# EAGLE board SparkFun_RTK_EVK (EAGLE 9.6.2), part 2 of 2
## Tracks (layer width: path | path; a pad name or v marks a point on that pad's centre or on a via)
3.3_SW
  cutout Route15: 93.54,72.77 93.41,72.77 93.03,72.39 93.03,69.72 93.66,69.09 94.68,68.07 95.95,68.07 96.96,67.06 96.96,65.79 96.96,55.63 97.73,54.86 98.49,54.1 101.03,54.1 106.11,54.1 106.62,53.59 128.46,31.75 129.22,31.75 129.73,31.75 130.11,32.13 130.11,32.77 129.6,33.27 129.22,33.27 106.87,55.63 105.09,55.63 99.25,55.63 98.74,56.13 98.49,56.39 98.49,57.91 98.49,67.82 97.47,68.83 96.58,69.72 95.82,69.72 95.19,69.72 94.81,70.1 94.68,70.23 94.68,70.99 94.68,72.01 94.17,72.52 93.92,72.77
3.3V  (via drill 0.3)
  Top 0.406: C25.1 v68.9,24.77 | C26.1 v70.55,24.77 | v72.71,24.64 U9.14 v72.71,26.67 | C1.1 87.74,29.63 R3.2 | VID2.1 92.56,29.63 v92.52,29.59 | v108.27,28.07 108.27,27.09 C3.1 C4.1 108.31,24.42 v108.27,24.38 U2.16 | U2.4 v112.08,18.8 | v82.99,31.37 83.97,31.37 C2.1 84.05,31.37 v85.03,31.37 86,31.37 C1.1 | C1.1 85.86,31.51 U1.2
  Top 0.61: U6.5 52.7,26.77
  Top 0.813: 52.7,26.77 C14.1 C15.1 52.6,23.71 3V3.1
  Route15 0.61: v72.71,24.64 72.71,24.77
  Route15 0.813: 3V3.1 53.02,22.86 55.69,25.53 65.85,25.53 66.61,24.77 v68.9,24.77 v70.55,24.77 72.71,24.77 v72.71,26.67 77.28,26.67 81.98,31.37 v82.99,31.37 90.74,31.37 v92.52,29.59 106.74,29.59 v108.27,28.07 v108.27,24.38 108.27,19.68 109.16,18.8 v112.08,18.8
  Bottom 0.152: I2C.2 75.88,21.46 v72.71,24.64
  cutout Route15: 22.8,91.06 arc-90 24.7,89.15 arc-90 22.8,87.25 arc-90 20.89,89.15 arc-90
3.3V_SW  (via drill 0.3)
  Top 0.152: U15.23 133.03,20.49 v132.99,20.45
  Top 0.305: v129.1,23.62 U15.15 | v136.97,22.1 136.44,22.63 U15.29 | U15.36 136.94,26.13 v136.97,26.16 | v132.98,28.07 v132.99,28.07 133.03,28.02 U15.5 | U15.10 129.13,26.13 v129.1,26.16 | U7.28 59.73,73.68 v59.75,73.66
  Top 0.406: C32.1 v59.75,73.66
  Top 0.61: U3.5 57.78,27.53 | 3V3_SW.1 58.1,22.86 58.1,19.05 63.69,13.46 76.38,13.46 | J4.2 76.38,13.46 | C56.1 81.34,14.35 80.45,13.46 76.38,13.46
  Top 0.813: 57.78,27.53 C6.1 C7.1 57.68,24.98 3V3_SW.1 50.9,18.2 C19.1 C20.1 C18.1 | J3.4 46.89,13.88 46.42,14.35 C18.1 | C18.1 45.81,18.2 44.11,19.9 R11.2 R65.2 | v124.52,24.51 R18.2 | C5.1 v76.77,66.55 | C62.1 v76.77,64.9 v76.77,66.55 | U5.22 78.58,68.86 78.58,67.91 78.42,67.76 | v41.48,88.39 C52.1 | C55.1 v41.48,86.74 v41.48,88.39 | R30.2 v51.75,84.58 | R31.2 v53.53,84.58 | R32.2 v55.31,84.58 | C21.1 C32.1 | FB2.1 v43.37,67.31 v42.74,67.31 | R64.2 v76.77,75.18 | R28.2 104.2,82.46 104.46,82.21 v104.46,82.17 | v115.13,82.17 v113.47,82.17 C29.1 | v116.78,82.17 v115.13,82.17 | C30.1 v115.13,82.17 | C24.1 v116.78,82.17 | U4.36 118.68,72.14 | 118.68,72.14 118.68,74.3 | 118.68,74.3 118.68,81.28 117.79,82.17 v116.78,82.17 | U4.38 118.64,74.33 118.68,74.3 | U4.33 118.3,68.83 118.68,69.22 118.68,69.98 | 118.68,69.98 118.68,72.14 | U4.34 118.64,69.94 118.68,69.98 | R57.1 v72.83,46.61 | R54.1 69.91,39.79 v69.91,40.89 | v76.77,66.55 77.98,67.76 78.42,67.76 | 78.42,67.76 U5.23 | v96.71,73.28 95.61,73.28 C12.1 92.06,73.24 U5.7 | J13.7 41.48,95.56 v41.48,88.39
  Bottom 0.152: I2C1.2 v110.17,86.49
  pour Route15 (isolate 0.203, rank 3): 4.76,0 4.76,50.42 17.59,50.42 18.1,50.93 18.73,51.56 18.73,52.45 18.73,78.87 17.34,80.26 14.92,82.68 14.92,83.82 14.92,84.2 14.41,84.71 13.65,85.47 13.65,90.04 13.65,93.09 12.26,94.49 11.62,95.12 8.45,95.12 4.76,95.12 4.76,101.6 147,101.6 147,0
  cutout Route15: 118.43,75.95 118.43,76.58 118.05,76.96 117.54,76.96 117.28,76.71 113.35,72.77 113.35,71.37 113.35,50.04 116.27,47.12 131.64,31.75 132.02,31.75 133.03,31.75 133.41,32.13 133.41,32.77 132.78,33.4 132.65,33.53 132.52,33.53 115.13,50.93 115.13,52.2 115.13,72.01 115.89,72.77 118.43,75.31
  cutout Route15: 133.03,59.31 132.65,59.31 132.27,58.93 132.27,58.42 132.91,57.78 134.43,56.26 134.43,55.37 134.43,32.13 134.81,31.75 136.21,31.75 136.46,31.75 136.84,32.13 136.84,32.89 136.46,33.27 136.46,33.91 136.46,57.28 135.7,58.04 134.43,59.31
3.3V_SW2  (via drill 0.3)
  Top 0.152: U16.15 121.96,46.89 122.62,46.23 126.68,46.23 127.06,46.61 127.06,52.45 127.95,53.34 130.49,53.34 131.14,53.99 U18.5 134.07,54.93 135.41,53.59 v140.65,53.59
  Top 0.406: U12.1 60.94,28.41 61.02,28.32
  Top 0.813: 3V3_SW2.1 61.06,23.71 C61.1 C60.1 61.06,28.28 61.02,28.32 | v141.92,53.59 v140.65,53.59 | v141.92,53.59 v143.19,53.59 | 140.14,82.3 140.14,83.19 139.94,83.39 U8.53 C80.1 C79.1 138.75,88.94 C81.1 140.44,88.9 C78.1 142.04,88.85 C77.1 141.92,87.01 C76.+ v141.92,53.59 | 140.14,82.3 140.14,81.41 139.93,81.19 U8.51 | U8.52 140.14,82.29 140.14,82.3
  Route15 0.813: v140.65,53.59 v141.92,53.59 v143.19,53.59 144.46,52.32 144.46,20.32 140.65,16.51 126.68,16.51 122.62,12.45 108.52,12.45 106.36,14.61 99.38,14.61 91.16,22.82 61.95,22.82 3V3_SW2.1
5V
  Top 0.152: U6.3 50.8,32.96 51.24,33.4 52.7,33.4
  Top 0.406: U12.8 60.94,32.55 61.02,32.64
  Top 0.61: U6.1 52.7,33.4 | U3.1 57.78,34.19
  Top 0.813: 52.7,33.4 52.7,34.19 C17.1 R51.2 R50.2 52.6,38.95 54.29,40.64 5V.1 | 57.78,34.19 C9.1 C8.1 C10.1 | 5V.1 57.68,40.22 C10.1 | C10.1 C23.1 C22.1 C59.1 61.06,32.68 61.02,32.64 | R59.1 F1.1 54.78,53.71 R53.1 | R59.1 57.97,48.13 56.69,46.85 C57.+ | C57.+ 56.69,43.32 58.1,41.91 5V.1 | 5V.1 58.14,40.68 60.26,40.68 C53.1 60.74,40.96 U13.5 | C57.+ 58.86,44.45 59.28,44.87 C54.1 60.74,44.77 U11.5 | R59.1 R55.1 R60.1 R61.1
5V_RAW
  Top 0.813: U10.2 U10.1 29.72,54.17 30.3,54.75 C48.+ 32.93,54.98 C49.1 | C49.1 C50.1 | L1.1 37.78,53.38 C49.1
5V_RAW1
  Top 0.813: C16.+ 41.96,26.9 C51.1 C84.1 42.06,33.63 L4.1
  Top 1.905: U17.4 C16.+
9%  (via drill 0.3)
  Top 0.152: 9%.1 50.48,58.42 53.87,58.42 | R48.2 53.87,58.42 | 53.87,58.42 R58.1 | U13.3 64.77,42.86 v63.94,43.69
  Bottom 0.152: v63.94,43.69 61.91,45.72 61.91,47.62 56.2,53.34 47.94,53.34 9%.1
99%  (via drill 0.3)
  Top 0.152: 99%.1 R53.2 R48.1 | U11.4 62.52,47.47 v62.55,47.5
  Bottom 0.152: v62.55,47.5 56.32,53.72 50.1,53.72 99%.1
!ANT_SHORT!  (via drill 0.3)
  Top 0.152: Q2.6 70.15,46.41 R57.2 69.95,47.41 ANT_SHT.1 | v78.6,48.26 78.72,48.39 v78.72,64.36 | v100.14,72.14 U4.6
  Bottom 0.152: ANT_SHT.1 v78.6,48.26 | v100.14,72.14 100.14,67.69 97.06,64.61 78.98,64.61 v78.72,64.36
!RESET!  (via drill 0.3)
  Top 0.152: U7.37 58.8,79.18 59.12,79.5 59.12,83.58 60.37,84.84 64.65,84.84 67.12,82.37 67.12,77.67 v67.32,77.47 67.12,77.27 67.12,57.02 v68.26,55.88 | v87.19,35.33 87.13,35.28 U1.3 87.13,32.95 87.95,32.13 R3.1 C31.1 91.12,30.06 91.12,27.94 v94.93,24.13 | U9.12 v75.25,35.31 74.87,35.69 v68.26,35.69 | v99.76,21.21 99.79,21.24 Q1.3
  Bottom 0.152: v67.32,77.47 GNSS_RESET.4 GNSS_RESET.2 | v87.19,35.33 75.28,35.33 v75.25,35.31 | v68.26,55.88 v68.26,35.69 | RESET_SW.1 101.28,12.7 98.74,15.24 98.74,20.19 v99.76,21.21 96.84,24.13 v94.93,24.13
!SAFEBOOT_NEO!
  Top 0.152: U5.1 94.06,66.66 94.68,66.04 !SAFEBOOT_NEO!.1
!SAFEBOOT_ZED!
  Top 0.152: U4.50 106.83,80.56 106.83,87.16 !SAFEBOOT_ZED!.1
ACT
  Bottom 0.152: ACT.1 9.07,98.16 8.29,97.38 J9.14
ACT_LED
  Top 0.152: U7.27 59.34,73.18 59.75,72.77 59.75,70.23 60.13,69.85 R26.2
ANT
  Top 0.349: C13.2 U14.2
ANT_DET  (via drill 0.3)
  Top 0.152: Q2.3 71.45,39.95 R54.2 71.65,38.95 ANT_DET.1 | v79.69,65.41 v79.69,38.1 | U4.4 100.05,74.33 99.63,73.91 v99.63,71.63
  Bottom 0.152: v99.63,71.63 99.63,67.7 96.82,64.89 80.2,64.89 v79.69,65.41 | v79.69,38.1 ANT_DET.1
ANT_NEO
  Top 0.318: 92.1,79.5 arc-90 U5.11
  Top 0.349: U14.5 94.93,81.03 arc-90 93.41,79.5 92.1,79.5
ANT_ZED
  Top 0.318: 101.41,76.58 arc-90 U4.2
  Top 0.349: U14.8 98.74,78.23 arc90 100.39,76.58 101.41,76.58
BYPASS
  Top 0.349: BYPASS1.1 97.47,85.72 arc90 98.11,85.09 arc-90 98.74,84.45 BYPASS2.1
CH340-DTR  (via drill 0.3)
  Top 0.152: R4.2 103.75,21.24 v102.81,21.24 Q1.1 101.93,22.21 101.28,22.86 DTR.1 | U2.13 112.08,21.84 111.44,21.21 v106.36,21.21
  Bottom 0.152: v106.36,21.21 102.84,21.21
  Bottom 0.267: 102.84,21.21 v102.81,21.24
CH340-RTS  (via drill 0.3)
  Top 0.152: R5.2 98.81,19.4 v99.76,19.4 Q1.4 100.63,18.43 101.28,17.78 RTS.1 | U2.14 110.81,22.23 110.43,21.85 105.99,21.85 105.22,21.08 v105.22,19.43
  Bottom 0.152: 105.19,19.4 v99.76,19.4
  Bottom 0.267: v105.22,19.43 105.19,19.4
CH340-RXI  (via drill 0.3)
  Top 0.152: TX.1 110.81,15.88 U2.3 v110.81,19.94 | v94.93,47.62 94.81,47.5 92.7,47.5 88.4,51.8 U1.35
  Bottom 0.152: v110.81,19.94 109.28,19.94 109.03,20.19 109.03,35.01 96.41,47.62 v94.93,47.62
CH340-TXO  (via drill 0.3)
  Top 0.152: RX.1 109.54,15.88 U2.2 v109.54,20.57 | v94.93,48.54 92.93,48.54 89.67,51.8 U1.34
  Bottom 0.152: v109.54,20.57 109.54,34.9 95.89,48.54 v94.93,48.54
D+  (via drill 0.3)
  Top 0.152: 113.73,8.89 J1.A6 113.73,5.33 113.98,5.08 114.49,5.08 114.73,5.32 J1.B6
  Top 0.267: 113.73,8.89 113.03,9.59 D10.1 113.03,11.37 v113.22,11.56 | v113.47,16.51 113.47,16.63 113.35,16.76 U2.5
  Bottom 0.267: v113.47,16.51 113.73,16.26 113.73,12.06 v113.22,11.56
D+_LARA
  Top 0.267: U15.2 134.53,27.79 135.19,28.45 135.19,29.25 R10.1
D+_NEO
  Top 0.267: R66.1 128.59,29.25 128.59,29.08 129.86,27.81 131.64,27.81 132.03,27.42 U15.7
D+_UBLOX
  Top 0.267: J6.A6 139.13,5.2 139.26,5.08 139.89,5.08 140.13,5.32 J6.B6 140.13,7.87 141.54,9.28 141.54,10.79 140.33,12 D8.1 140.33,13.15 139.92,13.56 139.92,15.31 R23.1
D+_ZED
  Top 0.267: R7.1 131.51,29.46 132.37,28.6 133.38,28.6 133.53,28.46 U15.4
D-  (via drill 0.3)
  Top 0.152: J1.B7 113.22,6 v113.22,7.11 | 114.23,8.89 114.23,7.24 v114.36,7.11 114.23,6.98 J1.A7
  Top 0.267: 114.23,8.89 114.93,9.59 D10.3 114.93,11.37 v114.74,11.56 | v114.49,16.51 114.62,16.64 U2.6
  Bottom 0.152: v114.36,7.11 v113.22,7.11
  Bottom 0.267: v114.49,16.51 114.24,16.26 114.24,12.06 v114.74,11.56
D-_LARA
  Top 0.267: U15.1 135.03,27.65 135.7,28.32 135.7,28.87 R9.1
D-_NEO
  Top 0.267: U15.6 132.53,27.53 131.85,28.21 130.1,28.21 129.48,28.83 129.48,29.25 R67.1
D-_UBLOX
  Top 0.267: J6.A7 139.63,6.99 | 139.63,6.99 139.63,8 141.02,9.38 141.02,10.76 140.1,11.68 138.62,11.68 138.43,11.87 D8.3 138.43,13.15 138.85,13.56 138.85,15.31 R22.1 | J6.B7 138.63,6.74 138.87,6.99 139.63,6.99
D-_ZED
  Top 0.267: U15.3 134.03,28.76 R8.1
ESP0/!BOOT!  (via drill 0.3)
  Top 0.152: Q1.6 101.93,18.89 102.03,18.8 v102.55,18.8 | U1.25 101.1,42.09 v101.28,41.91
  Bottom 0.152: v102.55,18.8 105.35,18.8 105.85,19.3 107.63,19.3 | 107.63,19.3 120.08,19.3 TP_BOOT.1 BOOT_SW.1 | v101.28,41.91 101.66,41.91 107.63,35.94 107.63,19.3
ESP2/LED  (via drill 0.3)
  Top 0.152: R62.1 TP_LED.1 | v98.74,62.28 98.74,59.44 99.76,58.42 101.92,58.42 102.37,57.97 U1.24
  Bottom 0.152: TP_LED.1 14.92,13.97 14.92,17.78 20,22.86 25.97,22.86 26.5,23.39 26.5,45.03 34.12,52.65 34.12,60.15 36.05,62.08 98.54,62.08 v98.74,62.28
ESP4/!SD_CS!  (via drill 0.3)
  Top 0.152: J3.2 49.09,13.85 SD_CS.1 | U1.26 99.83,56.47 v99.76,56.54 | v76.42,28.45 76.39,28.48 76.39,55.88 76.39,56.26 76.39,56.52 v76.14,56.77 | v66.99,28.45 v66.99,16.38
  Bottom 0.152: v76.42,28.45 v66.99,28.45 | v99.76,56.54 99.66,56.64 77.66,56.64 77.28,56.26 76.64,56.26 v76.14,56.77 | v66.99,16.38 51.63,16.38 SD_CS.1
ESP5/TP
  Top 0.152: U9.8 80.33,27.3 82.23,29.21 82.23,39.37 88.58,45.72 94.93,45.72 96.02,46.81 U1.29
ESP12/SDA2
  Top 0.152: U9.4 76.52,18.92 77.03,18.41 90.49,18.41 101.1,29.03 U1.14
ESP13/LARA_TXDI  (via drill 0.3)
  Top 0.152: U1.16 103.64,36.9 104.2,37.47 v119.82,37.47 119.82,36.2 119.57,35.94 119.44,35.94 119.06,35.56 119.06,30.48 TXD.1 | v119.95,46.48 119.95,47.84 U16.12
  Bottom 0.152: v119.82,37.47 119.82,46.35 v119.95,46.48
ESP14/LARA_RXDO  (via drill 0.3)
  Top 0.152: U1.13 99.83,36.9 100.9,37.97 120.46,37.97 v120.59,37.85 120.59,32 RXD.1 | v120.71,46.48 120.71,47.84 U16.13
  Bottom 0.152: v120.59,37.85 120.59,46.35 v120.71,46.48
ESP15/SCL2  (via drill 0.3)
  Top 0.152: U1.23 103.64,56.7 v103.57,56.77 | v76.9,56.77 v76.9,27.94 | v73.34,27.94 73.34,22.86 72.71,22.23 U9.1
  Bottom 0.152: v103.57,56.77 103.31,57.02 77.15,57.02 v76.9,56.77 | v76.9,27.94 v73.34,27.94
ESP18/SCK  (via drill 0.3)
  Top 0.152: J3.5 45.79,13.58 SCK.1 | U7.33 59.85,76.18 60.24,76.57 60.24,83.05 60.91,83.72 64.19,83.72 66,81.9 66,54.08 v66.23,53.85 66.3,53.78 v75.25,53.78 | v65.98,15.42 v65.98,30.1 | v94.68,53.72 94.75,53.65 U1.30
  Bottom 0.152: SCK.1 45.68,13.69 51.87,13.69 53.6,15.42 v65.98,15.42 | v65.98,30.1 66.02,30.1 66.2,30.28 66.2,53.82 v66.23,53.85 | v75.25,53.78 75.37,53.65 94.55,53.65 94.65,53.75 v94.68,53.72
ESP19/POCI  (via drill 0.3)
  Top 0.152: J3.7 43.59,13.49 41.85,15.24 POCI.1 41.59,16.3 R11.1 | U7.34 59.8,76.68 59.96,76.83 59.96,83.16 60.79,84 64.3,84 66.28,82.02 66.28,54.76 v66.71,54.33 74.54,54.33 v74.61,54.26 | v65.47,14.94 v65.47,28.83 | v93.41,54.23 93.48,54.16 U1.31
  Bottom 0.152: POCI.1 43.47,13.36 44.84,13.36 44.89,13.41 51.98,13.41 53.52,14.94 v65.47,14.94 | v65.47,28.83 65.47,28.91 66.71,30.15 v66.71,54.33 | v74.61,54.26 93.38,54.26 v93.41,54.23
ESP21/SDA  (via drill 0.3)
  Top 0.152: U5.18 80.01,73.23 v78.55,73.23 | v68.74,56.36 67.4,57.71 67.4,72.44 v67.6,72.64 67.88,72.93 67.88,82 64.03,85.85 47.18,85.85 44.92,88.11 44.92,92.02 | U4.44 113.3,81.33 113.09,81.53 112.46,81.53 111.06,82.93 R72.1 112.17,83.61 v112.2,83.57 | v90.87,63.22 v90.87,55.5 90.94,55.42 U1.33 90.94,51.8 93.21,49.53 v94.93,49.53
  Top 0.305: D15.1 44.92,92.02 J13.6
  Bottom 0.152: SDA.1 44.92,97.31 J13.6 | v67.6,72.64 77.96,72.64 v78.55,73.23 | v68.74,56.36 75.4,56.36 76.13,55.63 90.74,55.63 v90.87,55.5 | v112.2,83.57 112.2,82.93 108.42,79.15 108.42,73.92 97.84,63.35 91,63.35 v90.87,63.22 | USB251SDA.1 126.58,18.64 95.69,49.53 v94.93,49.53
ESP22/SCL  (via drill 0.3)
  Top 0.152: U5.19 78.57,72.16 v78.55,72.14 | v69.23,56.84 67.68,58.39 67.68,71.76 v67.97,72.05 68.16,72.24 68.16,82.12 64.15,86.13 49.7,86.13 48.42,87.4 48.42,92.02 | U4.45 112.2,81.28 111.82,81.66 109.92,81.66 109.41,82.17 R71.1 108.18,83.61 v108.14,83.57 | v88.33,63.5 88.33,57.43 v87.06,56.16 87.13,56.09 U1.36 87.13,51.87 89.47,49.53 v89.85,49.53
  Top 0.305: D16.1 48.42,92.02 J13.5
  Bottom 0.152: SCL.1 48.42,98.27 J13.5 | v67.97,72.05 68.28,72.36 77.81,72.36 78.04,72.14 v78.55,72.14 | v69.23,56.84 75.38,56.84 76.32,55.91 77.43,55.91 77.79,56.26 86.96,56.26 v87.06,56.16 | v108.14,83.57 108.14,74.17 97.68,63.7 88.53,63.7 v88.33,63.5 | USB251SCL.1 134.05,18.14 133.82,17.91 126.92,17.91 95.81,49.02 90.36,49.02 v89.85,49.53
ESP23/PICO  (via drill 0.3)
  Top 0.152: J3.3 47.94,12.58 PICO.1 | U7.35 59.51,77.18 59.68,77.34 59.68,83.28 60.68,84.28 64.42,84.28 66.56,82.14 66.56,55.55 v67.25,54.86 73.92,54.86 v73.98,54.81 | v66.48,15.9 v66.48,29.21 | v85.79,54.74 85.86,54.66 U1.37
  Bottom 0.152: PICO.1 49.21,13.97 51.75,13.97 53.69,15.9 v66.48,15.9 | v66.48,29.21 67.25,29.97 v67.25,54.86 | v73.98,54.81 85.72,54.81 v85.79,54.74
ESP25/ZED_TXO  (via drill 0.3)
  Top 0.152: U4.42 116.63,80.44 v116.68,80.39 | v94.81,62.56 94.81,55.75 v96.58,53.98 | v96.58,50.29 97.98,50.29 98.74,49.53 98.74,40.01 96.02,37.28 U1.10
  Bottom 0.152: v116.68,80.39 116.68,80.28 116.75,80.21 116.75,64.12 114.98,62.36 100.03,62.36 99.35,63.04 95.29,63.04 v94.81,62.56 | v96.58,53.98 v96.58,50.29 96.58,49.4 97.09,48.9 105.73,48.9 ZED_TXO.1
ESP26/LARA_PWR_ON
  Top 0.152: U1.11 97.29,36.65 98.97,38.33 124.37,38.33 131.76,45.72 R70.1 R69.2
ESP27/!ETH_CS!  (via drill 0.3)
  Top 0.152: U7.32 59.74,75.68 60.52,76.45 60.52,82.93 61.02,83.44 64.07,83.44 65.72,81.79 v65.72,53.34 | v65.72,36.83 v75.25,36.83 | v98.49,36.83 98.49,34.25 U1.12 98.56,33.2 ETH_CS.1
  Bottom 0.152: v65.72,53.34 v65.72,36.83 | v75.25,36.83 v98.49,36.83
ESP32/PWREN  (via drill 0.3)
  Top 0.152: U9.11 76.52,25.91 78.68,28.07 v78.68,37.34 | v93.41,37.31 93.41,34.25 U1.8
  Bottom 0.152: v78.68,37.34 93.38,37.34 v93.41,37.31
ESP33/ZED_RXI  (via drill 0.3)
  Top 0.152: U4.43 114.4,81.34 114.62,81.56 116.62,81.56 v117.16,81.03 | U1.9 94.75,36.65 97.47,39.37 v97.47,49.53 | v97.47,53.98 95.57,55.88 95.57,61.95 v96.17,62.56
  Bottom 0.152: v117.16,81.03 117.16,64.14 115.1,62.08 99.78,62.08 99.1,62.76 98.38,62.76 98.23,62.61 96.23,62.61 v96.17,62.56 | v97.47,53.98 v97.47,49.53 107.63,49.53 ZED_RXI.1
ESP34/LARA_NI  (via drill 0.3)
  Top 0.152: U16.14 121.31,40.34 119.57,38.61 v98.11,38.61 | v91,37.85 90.94,37.79 U1.6
  Bottom 0.152: v91,37.85 91.76,38.61 v98.11,38.61
ESP35/VID
  Top 0.152: VID1.2 VID2.2 92.81,31.33 92.21,31.93 U1.7
ESP36/SD_DET  (via drill 0.3)
  Top 0.152: J3.9 41.39,12.9 DET.1 39.05,15.41 R65.1 | v69.02,35.18 64.96,31.11 v64.96,14.46 | U1.4 88.4,35.74 v88.33,35.81
  Bottom 0.152: DET.1 41.21,13.08 44.96,13.08 45,13.13 52.1,13.13 53.43,14.46 v64.96,14.46 | v69.02,35.18 69.66,35.81 v88.33,35.81
ESP39/!ETH_INT!  (via drill 0.3)
  Top 0.152: U7.36 58.95,77.68 59.4,78.13 59.4,83.46 60.49,84.56 64.53,84.56 66.84,82.25 66.84,56.29 v67.75,55.37 | v67.75,36.32 v75.88,36.32 | U1.5 89.67,36.27 v89.73,36.32
  Bottom 0.152: v75.88,36.32 v89.73,36.32 95.44,36.32 97.47,34.29 ETH_INT.1 | v67.75,55.37 v67.75,36.32
GND  (via drill 0.3)
  Top 0.305: v129.1,24.89 129.1,25.31 129.42,25.63 U15.11 131.53,25.63 U15.EP
  Bottom 0.152: SHLD1.1 113.97,3.68 v112.59,3.68 | SHLD2.1 139.27,3.81 v138.11,3.81
  other vias: 28.89,73.66 28.89,72.39 28.89,71.12 28.89,69.85 26.35,68.58 26.35,67.31 26.35,66.04 26.35,64.77 26.35,63.5 26.35,62.23 26.35,60.96 26.35,59.69 27.62,59.69 27.62,60.96 27.62,62.23 27.62,63.5 27.62,64.77 27.62,66.04 27.62,67.31 27.62,68.58 28.89,68.58 28.89,67.31 28.89,66.04 28.89,64.77 28.89,63.5 28.89,62.23 28.89,60.96 28.89,59.69 28.26,60.33 26.99,60.33 26.99,61.59 28.26,61.59 28.26,62.87 26.99,62.87 26.99,64.14 26.99,65.41 26.99,66.67 28.26,67.94 26.99,67.94 28.26,66.67 28.26,65.41 28.26,64.14 26.99,59.05 28.26,59.05 27.62,58.42 26.35,58.42 28.89,58.42 41.59,59.69 42.86,59.69 44.13,59.69 45.4,59.69 46.67,59.69 45.4,58.42 46.67,58.42 44.13,58.42 42.23,59.05 43.5,59.05 44.77,59.05 44.77,57.78 46.04,59.05 46.04,57.78 40.32,59.69 39.05,59.69 39.05,58.42 40.32,58.42 40.96,59.05 39.69,59.05 39.69,57.78 40.96,57.78 21.02,17.14 16.45,17.14 26.86,21.08 28.51,21.08 29.78,21.08 25.21,21.08 23.56,21.08 30.29,16 62.93,28.19 63.94,26.67 63.94,24.51 49.72,26.67 49.72,24.77 54.67,25.78 54.67,27.43 56.83,32.89 56.83,30.73 51.75,30.73 51.75,32.89 63.94,29.21 54.8,36.2 54.8,38.1 63.94,38.1 63.94,36.2 63.82,33.4 49.72,34.29 54.93,33.4 32.7,61.59 31.81,61.59 33.59,61.59 37.78,57.78 41.08,54.48 50.86,59.69 63.94,45.72 63.94,41.91 60.64,47.75 59.5,42.8 70.17,42.04 71.44,45.59 49.21,44.45 49.21,45.47 49.21,43.43 142.05,48.77 141.03,48.77 143.07,48.77 118.43,49.4 129.86,55.88 133.41,52.07 128.59,51.31 127.57,62.99 129.6,62.99 131.76,62.99 133.92,62.99 135.95,62.99 125.16,60.33 138.24,60.33 127.57,69.34 135.95,69.34 127.57,75.44 135.95,75.44 127.57,81.79 129.73,81.79 131.76,81.79 133.79,81.79 135.95,81.79 123.51,81.15 123.51,83.44 125.03,84.45 127.32,86.36 126.3,86.36 127.32,87.63 127.32,88.9 127.32,90.17 127.32,91.44 126.81,92.2 125.41,92.08 123.76,92.08 121.98,92.08 120.71,92.08 119.19,92.58 118.55,93.98 117.28,95.25 117.16,96.65 115.76,99.31 115.76,98.04 116.01,96.9 115.76,100.33 123.63,100.33 123.63,99.31 123.63,98.04 123.38,96.77 122.36,96.65 120.97,95.89 121.73,94.87 123.76,94.87 125.41,96.39 126.94,95.12 128.08,94.11 129.22,92.71 129.22,91.44 129.22,90.17 129.22,88.9 129.22,87.63 129.22,86.36 130.49,86.36 134.3,86.36 133.03,86.36 134.3,87.63 134.3,88.9 134.3,90.17 134.3,91.44 134.3,92.71 134.81,94.11 135.57,95.12 136.84,96.27 137.99,99.31 137.99,100.33 137.99,98.04 138.24,96.65 139.38,96.65 140.65,95.25 138.49,95.25 145.86,99.31 145.86,100.33 145.86,98.04 145.61,96.65 144.59,96.65 144.21,95.25 143.19,94.11 142.68,92.96 141.41,92.2 140.4,92.08 138.62,92.08 136.97,92.08 136.08,91.06 135.83,88.9 135.83,87.25 136.08,85.98 137.22,85.98 101.54,99.06 101.54,100.33 101.54,97.79 101.28,96.52 100.01,96.52 98.74,95.25 98.74,93.47 98.74,91.69 98.74,89.92 96.2,89.92 96.2,91.69 94.55,91.69 93.03,90.42 91.12,91.44 95.06,95.25 94.42,94.49 94.93,96.52 93.66,96.65 93.41,99.06 93.41,97.79 93.41,100.33 94.93,89.15 94.93,85.09 96.2,85.09 97.47,84.2 98.74,85.98 96.2,81.28 97.47,81.28 93.54,86.87 93.54,85.09 93.54,83.31 93.79,80.9 92.14,81.92 90.36,80.64 90.36,79.63 90.36,78.49 94.04,78.49 95.44,79.63 97.73,79.76 97.73,78.23 98.23,76.71 99.76,75.44 99.76,77.72 99.76,79.76 99.76,81.28 100.39,82.8 100.39,85.09 100.39,87.63 101.41,78.61 103.82,76.71 108.9,76.71 112.97,76.71 112.97,72.52 108.9,72.52 104.71,68.33 108.9,68.33 112.97,68.33 104.71,64.14 108.9,64.14 112.97,64.14 117.79,67.82 117.79,77.6 100.01,63.37 117.79,73.28 71.18,99.06 79.31,99.06 71.18,100.46 71.18,97.54 79.31,97.41 79.31,100.46 72.71,96.52 72.83,94.61 77.79,96.65 76.9,95.5 76.39,94.61 76.52,92.46 77.79,90.81 76.64,89.03 73.98,89.03 75.25,89.03 72.83,90.68 73.98,92.46 48.07,21.84 46.29,21.84 49.72,21.84 44.64,13.84 44.77,11.18 40.83,37.59 45.02,33.53 78.42,12.45 78.42,11.43 82.61,16.38 67.63,21.84 71.69,21.84 80.33,21.72 83.76,21.97 110.17,13.46 117.79,13.46 113.98,11.56 139.76,32.51 145.99,25.27 145.99,23.5 124.65,22.86 124.65,26.16 72.58,66.55 72.58,64.9 81.47,66.67 81.47,80.64 124.4,50.8 118.81,52.2 116.27,50.8 52.01,71.88 53.02,71.88 51.24,73.66 54.55,71.88 57.34,74.17 51.24,76.58 51.5,78.11 43.37,73.03 43.37,71.12 43.37,69.22 63.94,73.66 63.94,71.75 49.21,65.28 51.12,65.28 53.02,65.28 54.93,65.28 56.83,65.28 58.74,65.28 48.07,83.31 63.44,82.93 61.53,82.93 40.32,83.31 37.27,71.12 37.27,83.82 37.02,86.74 37.02,88.39 37.78,77.47 72.58,73.53 95.57,70.36 107.38,17.53 83.63,52.7 83.63,51.69 83.63,33.66 83.63,34.67 89.98,41.66 92.39,39.37 89.98,39.37 92.39,44.07 89.98,44.07 94.81,41.66 94.81,44.07 94.81,39.37 102.43,35.43 95.57,28.45 89.85,28.45 86.04,28.45 84.01,28.45 135.57,13.46 143.19,13.46 139.38,13.97 117.28,6.99 108.52,5.97 142.68,6.99 133.92,5.97 130.11,14.48 131.76,14.48 133.41,14.48 136.72,14.48 138.11,32.51 55.56,59.69 55.56,57.15 55.56,54.61 56.32,52.07 56.32,49.53 63.18,59.69 63.18,57.15 69.53,60.45 73.34,60.45 77.15,60.45 82.23,60.45 84.77,60.45 70.8,58.67 73.34,58.67 75.88,58.67 78.17,58.67 81.6,58.67 83.5,58.67 86.04,58.67 84.77,63.37 87.31,60.45 87.31,63.37 84.77,67.31 87.31,67.31 87.31,69.85 84.77,69.85 84.77,72.39 84.77,74.93 84.77,78.74 84.77,81.28 87.31,72.39 87.31,74.93 87.31,78.74 87.31,81.28 84.77,83.82 84.77,86.36 84.77,88.9 84.77,91.44 86.04,93.98 88.58,94.61 91.12,94.61 87.31,83.82 87.31,86.36 87.31,88.9 88.58,91.44 103.82,74.68 103.82,78.87 100.01,64.77 135.57,58.67 123.51,69.09 145.1,88.9 144.97,87.12 108.9,81.79 113.47,86.61 115,86.61 116.78,86.61 140.02,80.01 123.51,78.99 123.51,74.55 123.51,73.53 140.02,72.39 123.51,62.48 111.32,27.05 111.32,25.4 106.87,76.71 104.71,72.64 128.46,14.48 126.81,14.48 46.67,89.79 50.23,89.79 53.66,89.79 57.21,89.79 60.64,89.79 64.33,89.79 125.41,55.88 133.03,24.13 84.77,48.26 86.04,48.26 14.92,87.63 17.46,87.63 14.92,90.17 23.81,83.82 32.7,83.82 31.43,74.93 26.35,74.93 26.35,77.47 31.43,77.47 28.89,77.47 20.89,80.64 19.62,78.23
  pour Top (isolate 0.203, rank 2): 4.76,0 4.76,50.42 17.59,50.42 18.73,51.56 18.73,78.85 14.88,82.7 14.88,84.3 13.65,85.47 13.65,93.09 11.62,95.12 4.76,95.12 4.76,101.6 147,101.6 147,0
  pour Bottom (isolate 0.203, rank 2): 4.76,0 4.76,50.42 17.59,50.42 18.73,51.56 18.73,78.85 14.88,82.7 14.88,84.3 13.65,85.47 13.65,93.09 11.62,95.12 4.76,95.12 4.76,101.6 147,101.6 147,0
  pour Route2 (isolate 0.203): 4.76,0 4.76,50.42 17.59,50.42 18.73,51.56 18.73,78.85 14.88,82.7 14.88,84.3 13.65,85.47 13.65,93.09 11.62,95.12 4.76,95.12 4.76,101.6 147,101.6 147,0
  cutout Top: 22.8,91.06 arc-90 24.7,89.15 arc-90 22.8,87.25 arc-90 20.89,89.15 arc-90
  cutout Bottom: 22.8,91.06 arc-90 24.7,89.15 arc-90 22.8,87.25 arc-90 20.89,89.15 arc-90
  cutout Route2: 22.8,91.06 arc-90 24.7,89.15 arc-90 22.8,87.25 arc-90 20.89,89.15 arc-90
  pour Top (isolate 0.127): 71.06,101.6 79.44,101.6 79.44,88.27 71.06,88.27
  cutout Route15 (isolate 0.203): 71.06,88.27 71.06,101.6 79.44,101.6 79.44,88.27
  cutout Route15 (isolate 0.203): 89.85,74.68 89.85,101.6 103.82,101.6 103.82,74.68
  cutout Route15 (isolate 0.203): 115.63,82.68 115.63,101.6 147,101.6 147,82.68
  pour Route15 (isolate 0.254, rank 2, no thermals): 13.65,88.9 20,88.9 24.96,83.95 53.02,83.95 53.02,68.2 29.4,68.2 14.92,82.68 14.92,84.2 13.65,85.41
GND-ISO  (1 unrouted)
  pour Top (isolate 0.406, rank 2): 4.76,93.85 11.11,93.85 12.38,92.58 12.38,84.96 13.68,83.7 13.68,82.2 17.46,78.42 17.46,52.32 16.7,51.56 4.76,51.56
  pour Route2 (isolate 0.203): 4.76,93.85 11.11,93.85 12.38,92.58 12.38,84.96 13.68,83.7 13.68,82.2 17.46,78.42 17.46,52.32 16.7,51.56 4.76,51.56
  pour Route15 (isolate 0.203): 4.76,93.85 11.11,93.85 12.38,92.58 12.38,84.96 13.68,83.7 13.68,82.2 17.46,78.42 17.46,52.32 16.7,51.56 4.76,51.56
  pour Bottom (isolate 0.406, rank 2): 4.76,93.85 11.11,93.85 12.38,92.58 12.38,84.96 13.68,83.7 13.68,82.2 17.46,78.42 17.46,52.32 16.7,51.56 4.76,51.56
GNSS_!RESET!  (via drill 0.3)
  Top 0.152: v93.66,76.2 92.1,76.2 U5.8 | GNSS_RESET.3 75.88,77.22 73.85,75.18 R64.1 74.61,74.33 74.61,74.13 C58.1 | U4.49 107.76,80.48 107.76,83.19 v107.38,83.57 | v98.23,72.77 98.23,58.8 98.87,58.17 v99,58.17 | v130.49,57.91 U18.2
  Bottom 0.152: GNSS_RESET.1 GNSS_RESET.3 77.15,76.2 v93.66,76.2 95.57,74.3 96.71,74.3 v98.23,72.77 103.82,72.77 104.97,73.91 104.97,83.31 102.17,86.11 102.17,86.61 102.55,87 104.58,87 106.36,85.22 106.36,83.82 106.62,83.57 v107.38,83.57 | v130.49,57.91 99.25,57.91 v99,58.17
LARA_18_NI
  Top 0.152: U16.3 121.31,54.84 121.43,54.97 121.43,64.73 123.6,66.89 U8.16
LARA_18_RXDO
  Top 0.152: U16.4 120.66,54.97 120.4,55.22 120.4,67.38 123.21,70.19 U8.13
LARA_18_TXDI
  Top 0.152: U16.5 120.01,67.49 123.8,71.29 U8.12
LARA_!RESET!
  Top 0.152: U8.18 122.79,64.69 122.24,64.14 122.24,56.77 124.05,54.95 Q6.3
LARA_PWR_ON  (via drill 0.3)
  Top 0.152: U8.15 122.28,67.99 120.97,66.67 120.97,56.6 v120.88,56.52 | Q5.3 128.55,49.28 v127.57,49.28
  Bottom 0.152: v120.88,56.52 123.51,56.52 127.57,52.45 v127.57,49.28
LINK
  Bottom 0.152: LINK.1 20.78,97.42 20.38,97.03 19.78,97.03 J9.12
LINK_LED
  Top 0.152: U7.25 58.54,70.47 R25.2
MEAS
  Top 0.813: MEAS.4 46.55,50.68 D9.C D5.C D6.C D4.C
  Bottom 0.152: MEAS.4 MEAS.2
N$1
  Top 0.152: J1.B5 115.73,8.52 R1.2
N$2
  Top 0.152: J1.A5 112.73,8.02 R2.2
N$3  (via drill 0.3)
  Top 0.267: R7.2 131.76,31.58 v131.76,32.51 | v117.79,76.33 116.56,76.33 U4.40
  Route15 0.267: v131.76,32.51 113.98,50.29 113.98,72.52 v117.79,76.33
N$4
  Top 0.152: Q1.2 101.28,22.23 101.03,22.48 99,22.48 98.74,22.23 R5.1
N$5
  Top 0.152: Q1.5 101.28,18.54 101.54,18.29 103.7,18.29 103.82,18.41 R4.1
N$6  (via drill 0.3)
  Top 0.267: R8.2 132.78,31.71 v132.78,32.51 | v117.79,75.44 U4.39
  Route15 0.267: v132.78,32.51 132.27,33.02 132.02,33.02 114.49,50.55 114.49,72.26 117.67,75.44 v117.79,75.44
N$7  (via drill 0.3)
  Top 0.152: R62.2 9.84,12.7 8.57,11.43 8.57,5.08 v9.84,3.81
  Bottom 0.152: v9.84,3.81 10.48,3.17 LED.2
N$8
  Bottom 0.152: J6.SHLD1 J6.SHLD3 139.38,1.25 | 139.38,1.25 J6.SHLD4 J6.SHLD2 | SHLD2.2 139.38,1.25
N$9
  Top 0.152: U4.51 105.6,81.92 105.85,82.17 R27.1
N$10
  Top 0.813: MEAS.3 F1.2
  Bottom 0.152: MEAS.3 MEAS.1
N$11
  Top 0.152: U4.27 115.5,59.06 115.76,58.8 R46.1
N$12  (via drill 0.3)
  Top 0.152: R26.1 v63.94,69.85
  Bottom 0.152: v63.94,69.85 60.64,69.85 53.02,77.47 49.21,77.47 41.21,85.47 23.43,85.47 17.46,91.44 17.46,96.52 15.56,98.42 ACT.2
N$13
  Top 0.318: ESP32_RF.SIG 75.25,94.67 D3.1 75.19,92.44 J8.FEED
N$14  (via drill 0.3)
  Top 0.152: R16.2 71.78,17.36 v70.8,16.38
  Bottom 0.152: v70.8,16.38 71.44,17.02 74.23,17.02 75.07,16.18 I2C.3
N$15  (via drill 0.3)
  Top 0.152: R19.2 79.36,17.36 v78.42,16.42
  Bottom 0.152: v78.42,16.42 78.42,15.75 77.91,15.24 I2C.1
N$16
  Top 0.152: U18.4 128.05,54.93 R68.1
N$17  (via drill 0.3)
  Top 0.267: v128.46,32.51 128.46,31.58 R66.2 | v93.54,72.14 92.07,72.14 U5.6
  Route15 0.267: v128.46,32.51 106.36,54.61 98.74,54.61 97.47,55.88 97.47,67.31 96.2,68.58 94.93,68.58 93.54,69.98 v93.54,72.14
N$18  (via drill 0.3)
  Top 0.267: U5.5 94.1,71.06 v94.17,70.99 | v129.48,32.51 129.48,31.71 R67.2
  Route15 0.267: v94.17,70.99 94.04,70.87 94.04,70.1 95.06,69.09 96.46,69.09 97.98,67.56 97.98,56.13 99,55.12 106.62,55.12 129.22,32.51 v129.48,32.51
N$19
  Top 0.152: U7.31 60.1,75.18 Y1.1 61.67,78.33 R24.1 61.7,80.01 C27.1
N$20
  Top 0.152: U7.30 60.13,74.68 62.42,74.68 62.67,74.92 Y1.3 63.35,76.08 63.35,78.31 R24.2 63.4,80.01 C28.1
N$21  (via drill 0.3)
  Top 0.152: v17.46,97.79 v16.19,96.52 | v63.94,67.94 R25.1
  Bottom 0.152: LINK.2 18.1,98.42 v17.46,97.79 | v16.19,96.52 16.19,92.2 23.33,85.06 41.11,85.06 48.98,77.19 52.91,77.19 62.15,67.94 v63.94,67.94
N$22  (via drill 0.3)
  Top 0.152: v49.72,38.1 R50.1
  Bottom 0.152: v49.72,38.1 53.02,38.1 54.29,36.83 54.29,34.92 54.93,34.29 SPWR.3
N$23
  Top 0.152: R29.2 46.41,73.18 U7.10
N$24
  Top 0.152: U7.22 56.04,69.88 56.83,69.09 C40.1
N$25
  Top 0.152: U7.20 55.04,69.97 54.67,69.6 54.42,69.6 53.02,68.2 C41.1
N$26  (via drill 0.3)
  Top 0.152: v55.94,32.89 55.94,31.84 U3.3
  Bottom 0.152: v55.94,32.89 56.15,32.89 56.83,33.57 SPWR.2
N$27
  Top 0.61: LOAD.1 R45.2
N$28
  Bottom 0.152: RESET_SW.2 101.28,6.06 RESET.2
N$29
  Bottom 0.152: BOOT.2 126.68,5.17 BOOT_SW.2
N$30
  Top 0.152: U7.23 56.54,69.77 56.97,69.34 57.56,69.34 R49.2
N$31  (via drill 0.3)
  Top 0.152: v49.72,36.2 R51.1
  Bottom 0.152: TPWR.3 60.87,32.87 59.88,31.88 54.8,31.88 53.78,32.89 53.78,35.56 53.15,36.2 v49.72,36.2
N$32
  Top 0.152: U4.26 114.4,59.09 114.11,58.8 R47.1
N$33
  Top 0.152: R33.2 143.19,9.53 142.56,8.89 142.05,8.89 141.13,7.97 J6.B5
N$34
  Top 0.152: J6.A5 138.13,8.02 R34.2
N$35
  Top 0.152: U11.1 67.53,44.77 R56.1
N$36
  Top 0.152: U4.53 103.4,81.7 102.55,82.55 R6.1
N$38
  Top 0.152: R56.2 69.02,45.17 69.02,44.32 69.41,43.94 70.55,43.94 70.8,44.2 Q2.5
N$39  (via drill 0.3)
  Top 0.152: v62.42,32.77 62.89,32.3 U12.5
  Bottom 0.152: TPWR.2 61.91,33.27 v62.42,32.77
N$40
  Top 0.152: R63.2 68.86,41.53 70.42,41.53 70.8,41.91 Q2.2
N$41
  Top 0.152: U13.1 67.53,40.96 R63.1
N$42
  Top 0.152: Q6.1 127.88,56.8 R68.2
N$43  (via drill 0.3)
  Top 0.152: R71.2 v109.41,86.49
  Bottom 0.152: v109.41,86.49 109.36,86.54 I2C1.3
N$44  (via drill 0.3)
  Top 0.152: R72.2 v111.06,86.49
  Bottom 0.152: v111.06,86.49 110.99,86.56 I2C1.1
N$45
  Bottom 0.152: LED.1 12.9,4.56 11.83,5.63 D2.A
N$46  (via drill 0.3)
  Top 0.267: R9.2 136.08,31.71 v136.08,32.51 | v133.03,58.67 133.03,60.27 U8.28
  Route15 0.267: v136.08,32.51 135.7,32.89 135.7,57.02 134.05,58.67 v133.03,58.67
N$47  (via drill 0.3)
  Top 0.267: R10.2 135.19,31.71 v135.19,32.51 | v133.79,58.04 133.79,60.27 U8.29
  Route15 0.267: v135.19,32.51 135.19,56.9 134.05,58.04 v133.79,58.04
N$48
  Top 0.152: 139.76,25.49 137.77,25.49 136.91,24.63 U15.33 | 139.76,25.49 141.03,25.49 R13.2 141.33,25.27 C63.2 | Y2.3 139.68,25.4 139.76,25.49
N$49
  Top 0.152: U15.32 136.97,24.13 137.77,23.33 138.24,23.33 | 138.24,23.33 141.08,23.33 R13.1 141.33,23.5 C64.2 | Y2.1 138.33,23.42 138.24,23.33
N$50
  Top 0.152: R12.1 138.11,26.63 137.12,25.63 U15.35
N$51
  Top 0.152: U15.28 135.78,21.25 136.72,20.32 R14.2
N$52
  Top 0.152: R17.2 130.11,18.67 130.49,19.05 133.54,19.05 134.16,19.67 134.16,20.68 134.03,20.81 U15.25
N$53
  Top 0.152: C65.1 139.76,27.88 137.01,25.13 U15.34
N$54
  Top 0.152: C66.1 128.46,25.23 128.46,24.51 128.84,24.13 U15.14
N$55
  Top 0.267: U15.30 136.83,23.13 139.13,20.83 139.13,18 R22.2
N$56
  Top 0.267: U15.31 136.96,23.63 139.64,20.95 139.64,18 R23.2
N$61
  Top 0.318: 141.92,95.19 arc-90 D12.1
  Top 0.349: C82.2 141.29,93.34 arc90 141.92,93.98 141.92,95.19 | D12.1 arc-90 141.92,95.31 LARA_RF1.SIG
N$62
  Top 0.318: 138.49,93.38 arc-90 C82.1
  Top 0.349: U8.56 135.06,92.33 arc-90 136.12,93.38 L2.1 138.49,93.38
N$63
  Top 0.349: LARA_RF2.SIG 119.7,95.31 arc-90 D13.1 119.64,94.54 arc90 120.84,93.34 C83.2
N$64
  Top 0.318: 125.45,93.34 arc-90 L3.1 125.37,93.34
  Top 0.349: U8.62 128.46,91.56 arc90 126.68,93.34 125.45,93.34 | 125.37,93.34 C83.1
N$65
  Top 0.152: Q5.1 131.69,50.45 R70.2
NEO_RXI
  Top 0.152: U5.21 74.72,69.96 NEO_RX.1
NEO_TXO
  Top 0.152: U5.20 73.4,71.06 NEO_TX.1
PMODE0  (via drill 0.3)
  Top 0.152: U7.45 53.04,79.78 51.75,81.06 R30.1 51.71,81.66 50.74,81.66 50.48,81.41 v50.48,80.9
  Bottom 0.152: v50.48,80.9 51.12,80.9 51.5,81.28 PM0.2
PMODE1  (via drill 0.3)
  Top 0.152: U7.44 53.53,79.19 R31.1 52.81,81.7 52.64,81.53 v52.64,80.9
  Bottom 0.152: v52.64,80.9 53.15,80.9 53.53,81.28 PM1.2
PMODE2  (via drill 0.3)
  Top 0.152: U7.43 54.04,79.8 55.31,81.06 R32.1 56.29,81.7 56.58,81.41 v56.58,80.9
  Bottom 0.152: v56.58,80.9 55.82,80.9 55.56,81.15 PM2.2
PW1+  (via drill 0.3)
  Top 1.905: PW+.3 9.84,72.9 | 9.84,72.9 9.84,70.36 9.91,70.29 U10.6 | U10.5 9.91,72.83 9.84,72.9
  Bottom 0.152: PW+.3 PW+.1
  other vias: 9.84,68.58 11.11,68.58 9.84,67.31 9.84,66.04 9.84,64.77 11.11,64.77 11.11,66.04 11.11,67.31 10.48,67.94 9.21,67.94 9.21,66.67 9.21,65.41 9.21,64.14 10.48,64.14 10.48,65.41 10.48,66.67
  pour Top (isolate 0.406): 8.95,71.12 11.49,71.12 11.49,63.75 8.95,63.75
  pour Bottom (isolate 0.406): 8.83,68.96 11.49,68.96 11.49,63.75 8.83,63.75
PW1-  (via drill 0.3)
  Top 0.152: v8.57,59.69 7.3,59.69
  Top 1.905: PW-.3 7.3,59.69 7.3,56.77 | 7.3,56.77 7.3,54.23 7.36,54.17 U10.8 | U10.7 7.36,56.71 7.3,56.77
  Bottom 0.152: PW-.3 PW-.1
  other vias: 8.57,62.23 9.84,62.23 11.11,62.23 9.84,60.96 8.57,60.96 8.57,58.42 9.84,58.42 11.11,58.42 11.11,59.69 9.84,59.69 11.11,60.96 10.48,61.59 9.21,61.59 10.48,60.33 9.21,60.33 9.21,59.05 10.48,59.05
  pour Top (isolate 0.406): 7.3,62.61 11.49,62.61 11.49,57.15 7.3,57.15
  pour Bottom (isolate 0.406): 8.19,62.61 11.49,62.61 11.49,58.04 8.19,58.04
PW+
  Bottom 0.152: PW+.4 PW+.2
  Bottom 1.905: J9.9 9.84,82.68 PW+.4
PW-
  Bottom 0.152: PW-.4 PW-.2
  Bottom 1.905: J9.10 7.3,83.95 PW-.4
PWREN  (via drill 0.3)
  Top 0.152: U9.10 77.79,24.13 | 77.79,24.13 77.79,23.62 | 77.79,23.62 77.79,21.59 | 77.79,21.59 U9.5 | 77.79,24.13 74.61,24.13 73.98,24.77 U9.13 73.98,28.19 73.6,28.57 72.96,28.57 72.58,28.19 v72.58,27.94 | U9.6 79.06,20.95 78.42,21.59 77.79,21.59 | PWREN.1 84.77,24.13 84.35,23.71 R15.2 77.88,23.71 77.79,23.62
  Bottom 0.152: v72.58,27.94 65.47,27.94 64.83,28.57 64.83,35.18 64.45,35.56 62.93,35.56 | TPWR.1 62.95,35.53 62.93,35.56 | SPWR.1 57.87,35.33 58.1,35.56 62.93,35.56
RCT  (via drill 0.3)
  Top 0.229: C43.1 R40.1 R35.1 v33.21,74.93
  Bottom 0.229: J9.5 23.18,75.69 32.45,75.69 v33.21,74.93
RD+  (via drill 0.3)
  Top 0.229: v33.21,76.83 C45.2
  Bottom 0.229: J9.3 18.1,82.42 23.81,76.71 33.08,76.71 v33.21,76.83
RD-  (via drill 0.3)
  Top 0.229: v33.08,69.22 C44.2
  Bottom 0.229: J9.6 15.56,84.58 16.32,84.58 16.95,83.95 16.95,82.8 23.56,76.2 34.86,76.2 35.75,75.31 35.75,69.98 34.99,69.22 v33.08,69.22
RF
  Top 0.318: 97.48,91.67 arc-90 C13.1 | FB1.2 97.42,93.54 | D1.1 97.47,95.31
  Top 0.349: FB1.2 97.48,91.67 | 97.42,93.54 D1.1 | 97.47,95.31 GNSS_RF.SIG
RXN
  Top 0.229: R39.1 47.41,75.68 U7.5
RXN1  (via drill 0.3)
  Top 0.229: R39.2 43.79,76.07 v43.37,76.07 42.92,76.52 D7.4 | v37.27,73.03 R40.2 | v37.27,69.22 C44.1
  Bottom 0.229: v43.37,76.07 43.24,76.2 37.4,76.2 36.51,75.31 36.51,73.79 v37.27,73.03 36.51,72.26 36.51,69.98 v37.27,69.22
RXP
  Top 0.229: R38.1 46.5,75.18 U7.6
RXP1  (via drill 0.3)
  Top 0.229: R38.2 44.17,75.31 v43.37,75.31 | D7.3 37.6,76.52 v37.4,76.72 36.21,76.72 C45.1 R35.2
  Bottom 0.229: v43.37,75.31 43.62,75.31 44.01,75.69 44.01,76.45 43.75,76.71 37.41,76.71 v37.4,76.72
SCL2  (via drill 0.3)
  Top 0.152: U9.2 v73.98,16.38 | v70.8,15.62 72.03,15.62 R16.1 | J4.4 73.2,11.93 72.71,11.43 SCL2.1
  Bottom 0.152: v73.98,16.38 71.56,16.38 v70.8,15.62 SCL2.1
SDA2  (via drill 0.3)
  Top 0.152: U9.3 75.25,18.41 78,15.66 78.42,15.66 | 78.42,15.66 R19.1 | J4.3 75.38,11.04 75.59,10.83 80.36,10.83 SDA2.1 | v78.42,14.68 78.42,15.66
  Bottom 0.152: SDA2.1 78.42,13.97 v78.42,14.68
SHIELD
  Bottom 0.152: J1.SHLD1 J1.SHLD3 113.98,1.25 | 113.98,1.25 J1.SHLD4 J1.SHLD2 | SHLD1.2 113.98,1.25
SIM_CLK  (via drill 0.3)
  Top 0.152: C71.1 23.81,17.95 v23.81,16.51 23.81,15.03 J2.C3 23.52,14.9 22.22,16.2 D11.1 | U8.38 140.11,66.89 v140.14,66.93
  Bottom 0.152: v140.14,66.93 141.03,66.93 142.28,65.68 142.28,62.5 141.58,61.8 36.17,61.8 34.4,60.04 34.4,52.53 26.78,44.91 26.78,22.42 26.07,21.71 26.07,18.77 v23.81,16.51
SIM_IO  (via drill 0.3)
  Top 0.152: D11.6 17.9,16.2 18.86,15.24 22.78,15.24 23.3,14.72 23.3,14.22 23.56,13.97 24.57,13.97 25.21,14.61 J2.C7 v25.21,16.51 C74.2 | U8.39 140.1,67.99 v140.14,67.94
  Bottom 0.152: v140.14,67.94 141.41,67.94 142.56,66.8 142.56,62.38 141.69,61.52 36.28,61.52 34.68,59.92 34.68,52.41 27.06,44.79 27.06,22.3 26.35,21.59 26.35,17.65 v25.21,16.51
SIM_RST  (via drill 0.3)
  Top 0.152: D11.4 16.25,18.09 15.94,17.78 15.94,16.38 17.36,14.96 22.67,14.96 23.03,14.6 23.03,14.11 23.44,13.69 25.57,13.69 26.48,14.61 J2.C2 26.35,15.03 v26.35,16.51 26.86,17.02 C72.2 | U8.40 v140.14,69.09
  Bottom 0.152: v140.14,69.09 141.41,69.09 142.91,67.59 142.91,62.35 141.81,61.24 36.4,61.24 34.96,59.81 34.96,52.3 27.34,44.68 27.34,17.5 v26.35,16.51
TCT  (via drill 0.3)
  Top 0.229: C46.1 R43.1 33.21,82.55 v33.08,82.68
  Bottom 0.229: J9.4 17.97,87 20,87 20.51,86.49 20.51,85.09 21.78,83.82 21.78,82.8 22.03,82.55 32.96,82.55 v33.08,82.68
TD+  (via drill 0.3)
  Top 0.229: D7.6 42.16,78.42 42.93,79.18 v43.31,79.18 44.07,79.18 44.51,78.74 R36.2 | v37.4,80.14 36.6,80.14 R41.1
  Bottom 0.229: v43.31,79.18 43.88,79.76 43.88,80.39 43.53,80.74 42.96,80.74 40.96,78.74 39.18,78.74 37.91,80.01 37.53,80.01 v37.4,80.14 37.15,80.14 35.24,82.04 21.02,82.04 20.64,82.42 J9.1
TD-  (via drill 0.3)
  Top 0.229: R37.2 44.04,80.14 v43.24,80.14 | R42.1 36.73,79.38 v37.4,79.38 37.66,79.38 38.61,78.42 D7.1
  Bottom 0.229: J9.2 19.49,85.72 19.49,82.8 20.76,81.53 34.99,81.53 37.02,79.5 37.27,79.5 v37.4,79.38 37.66,79.38 38.8,78.23 41.34,78.23 v43.24,80.14
TXN
  Top 0.229: R37.1 49.22,77.68 U7.1
TXP
  Top 0.229: R36.1 46.63,79.12 47.05,79.12 48.99,77.18 U7.2
USB251SCL  (via drill 0.3)
  Top 0.152: U15.24 133.53,20.58 v133.67,20.45 132.65,19.43 129.48,19.43 128.46,18.41 R52.2
  Bottom 0.152: v133.67,20.45 134.05,20.07 USB251SCL.2
USB251SDA  (via drill 0.3)
  Top 0.152: R44.2 126.81,18.29 128.33,19.81 131.51,19.81 v132.14,20.45 132.27,20.45 132.53,20.71 U15.22
  Bottom 0.152: USB251SDA.2 132.02,20.32 v132.14,20.45
USB_!RESET  (via drill 0.3)
  Top 0.152: R18.1 C67.1 127.57,22.86 v129.35,21.08 | U15.26 134.53,20.73 v134.94,20.32
  Bottom 0.152: v134.94,20.32 134.47,20.32 133.74,21.05 129.38,21.05 v129.35,21.08
V_ANT  (via drill 0.3)
  Top 0.152: R59.2 61.79,50.8 65.12,47.47 U11.3 64.13,46.67 63.44,45.97 63.44,43.05 63.24,42.86 U13.4
  Top 0.813: R59.2 R55.2 R60.2 R61.2 62.42,59.18 VANT.1 | FB1.1 93.07,93.47 C11.1 88.04,93.43 86.04,91.44 v86.04,59.56 v84.77,59.56
  Bottom 0.813: VANT.1 64.33,59.56 v84.77,59.56 v86.04,59.56
V_POE
  Top 0.61: LOAD.2 41.59,51.55
  Top 0.813: L1.2 38.19,51.68 C47.1 40.32,51.55 41.59,51.55 VPOE.1 D9.A
V_USB  (via drill 0.3, 0.5)
  Top 0.152: D10.5 113.98,13.72 114.24,13.97 115.25,13.97 115.76,13.46 115.76,9.05 v114.87,8.17
  Top 0.61: J1.VBUS2 116.43,7.53 v116.52,7.62 | J1.VBUS1 111.53,7.53 v111.44,7.62
  Top 0.813: D5.A VUSB.1
  Route15 0.813: v111.44,7.62 112.37,8.55 114.87,8.55 | 114.87,8.55 115.6,8.55 v116.52,7.62 115.98,8.17 v114.87,8.17 114.87,8.55
  Route15 1.905: VUSB.1 39.69,45.72 37.15,43.18 32.7,43.18 30.16,40.64 30.16,22.86 35.24,17.78 89.85,17.78 97.47,10.16 104.84,10.16 107.38,7.62 v111.44,7.62
V_USB_2  (via drill 0.3, 0.5)
  Top 0.152: v139.38,8.76 D8.5 139.38,10.92 139.13,11.18 137.86,11.18 136.59,12.45 136.59,13.21 135.06,14.73 R21.2 | U8.17 123.38,65.79 121.83,64.24 121.83,56.4 126.43,51.8 v126.43,46.92 | v145.73,46.99 145.73,26.21 146.47,25.47 146.47,23.3 145.73,22.56 145.73,9.53 143.83,7.62 v141.92,7.62
  Top 0.61: v141.92,7.62 141.83,7.53 J6.VBUS2 | J6.VBUS1 136.93,7.53 v136.84,7.62
  Top 0.813: D6.A VUSB2.1
  Route15 0.813: v136.84,7.62 137.99,8.76 v139.38,8.76 140.78,8.76 v141.92,7.62
  Route15 1.905: VUSB2.1 41.47,43.31 40.83,43.31 38.16,40.64 33.97,40.64 32.7,39.37 32.7,24.13 36.64,20.19 91.38,20.19 98.87,12.7 105.73,12.7 108.27,10.16 131.76,10.16 134.3,7.62 v136.84,7.62
  Bottom 0.152: v126.43,46.92 126.5,46.99 v145.73,46.99
VBUS_DET
  Top 0.152: U15.27 135.03,21.11 135.95,20.19 135.95,18.29 135.06,17.4 R21.1 R20.2 C68.1
VCCA  (via drill 0.3)
  Top 0.254: U7.4 50.02,76.2 v47.94,76.2 | U7.8 47.95,74.18 v47.94,74.17 | U7.11 47.98,72.68 v47.94,72.64 | v55.56,69.6 55.54,69.62 U7.21 | U7.17 v53.54,69.61 v53.53,69.6 | U7.15 52.54,69.62 v52.51,69.6
  Top 0.406: C33.1 54.93,69 55.54,69.62
  Top 0.61: v49.21,80.52 C38.1 | C39.1 v40.32,79.38 40.32,77.6 40.45,77.47 D7.5 | R41.2 33.34,80.64 33.08,80.39 v33.08,79.63 33.08,78.99 33.34,78.74 R42.2 | R43.2 v37.27,82.55
  Top 0.813: FB2.2 C36.1 | C36.1 C37.1 | C36.1 47.31,69.22 VCCA.1 47.94,69.43 C35.1 C34.1
  Route2 0.61: v33.08,79.63 36,82.55 v37.27,82.55 40.32,82.55 | 40.32,82.55 47.18,82.55 v49.21,80.52 47.94,79.25 v47.94,76.2 v47.94,74.17 v47.94,72.64 VCCA.1 48.2,69.6 v52.51,69.6 v53.53,69.6 v55.56,69.6 | v40.32,79.38 40.32,82.55
VCCIO
  Top 0.152: C69.1 122.63,47.92 U16.16 122.61,50.8 | U8.4 122.95,80.09 121.6,78.74 121.6,69.6 119.36,67.35 U16.6 119.36,50.84 119.32,50.8 | U16.1 122.61,50.8 | 119.32,50.8 118.68,50.8 118.06,51.42 U16.8 118.04,53.68 C70.1 113.05,53.68 112.71,53.34 VCCIO.1 | 119.32,50.8 121.98,50.8 | 121.98,50.8 122.61,50.8 | U16.2 121.96,50.83 121.98,50.8
VIN
  Top 0.813: L4.2 43.76,35.66 C85.1 44.25,38.08 D4.A VIN.1
VIN1+  (via drill 0.5)
  Top 1.905: v12.38,44.45 11.75,43.81 D14.A | v12.38,44.45 v12.38,43.18 11.74,43.18 D14.A | v12.38,44.45 11.74,44.45 D14.A
  Route2 1.905: VIN+.3 21.27,78.74 21.27,47.62 17.46,43.81 13.02,43.81 | 13.02,43.81 v12.38,44.45 | v12.38,43.18 13.02,43.81
  Bottom 0.152: VIN+.3 VIN+.1
VIN1-
  Top 1.27: C86.- 9.7,39.23 9.84,39.37
  Top 1.905: 9.84,39.37 U17.2
  Route2 1.905: U17.2 16.7,39.37 23.81,46.48 23.81,77.47 32.7,86.36 VIN-.4
  Bottom 0.152: VIN-.4 VIN-.2
VIN2+
  Top 1.905: D14.C 6.55,43.56 6.55,35.3 7.42,34.43 C86.+ 9.09,34.29 U17.3
VIN+
  Top 1.905: J13.10 30.92,92.2 30.16,91.44 VIN+.4
  Bottom 0.152: VIN+.4 VIN+.2
VIN-
  Top 1.905: J13.9 34.42,91.89 VIN-.3
  Bottom 0.152: VIN-.3 VIN-.1
VSIM  (via drill 0.3)
  Top 0.152: C75.2 C73.1 28.51,16.89 v28.89,16.51 28.89,15.03 J2.C1 | D11.3 20.95,18.09 v21.02,18.16 | v140.14,70.1 140.06,70.19 U8.41
  Bottom 0.152: v21.02,18.16 21.78,17.4 21.78,16.64 23.43,14.99 28.26,14.99 28.89,15.62 v28.89,16.51 27.62,17.78 27.62,44.45 35.24,52.07 35.24,59.69 36.51,60.96 141.92,60.96 143.19,62.23 143.19,68.58 141.67,70.1 v140.14,70.1
ZED_EXTINT  (via drill 0.3)
  Top 0.152: R27.2 R28.1 104.2,86.23 v104.08,86.36 | v69.28,63.32 69.02,63.57 69.02,82.44 64.49,86.97 60.03,86.97 58.92,88.08 58.92,92.02
  Top 0.305: D19.1 58.92,92.02 J13.2
  Bottom 0.152: ZED_EXTINT.1 58.92,96.97 J13.2 | v104.08,86.36 105.73,84.71 105.73,72.25 97.46,63.98 81.7,63.98 81.32,63.6 70.4,63.6 70.11,63.32 v69.28,63.32
ZED_RX2  (via drill 0.3)
  Top 0.152: v69.71,57.33 68.45,58.58 68.45,72.25 68.44,72.26 68.44,82.23 64.26,86.41 53.02,86.41 51.92,87.51 51.92,92.02 | v112.84,55.88 112.88,55.92 R47.2
  Top 0.305: D17.1 51.92,92.02 J13.4
  Bottom 0.152: RX2.1 51.92,98.89 J13.4 | v69.71,57.33 111.39,57.33 v112.84,55.88
ZED_TP  (via drill 0.3)
  Top 0.152: v102.81,86.36 102.81,85.56 R6.2 | v69.79,63.88 69.41,64.26 69.41,82.55 62.42,89.53 62.42,92.02 | U9.9 79.06,27.3 80.96,29.21 v80.96,64.14
  Top 0.305: D20.1 62.42,92.02 J13.1
  Bottom 0.152: TP.1 62.42,96.01 J13.1 | v102.81,86.36 105.35,83.82 105.35,72.39 97.22,64.26 81.22,64.26 81.09,64.14 v80.96,64.14 80.71,63.88 v69.79,63.88
ZED_TX2  (via drill 0.3)
  Top 0.152: v70.13,57.87 68.73,59.27 68.73,82.34 64.38,86.69 56.83,86.69 55.42,88.1 55.42,92.02 | v116.9,55.88 115.8,55.88 R46.2
  Top 0.305: D18.1 55.42,92.02 J13.3
  Bottom 0.152: TX2.1 55.42,97.93 J13.3 | v70.13,57.87 70.39,57.6 115.18,57.6 v116.9,55.88

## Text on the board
Top: 1
Route2: 2
Route15: 3
Bottom: v11 | 4
Measures: V-Score To V-Score | Dimensions / In Inches
tDocu: Controlled Impedance: JLC7628 / Material: TG155 / 4-Layers / Thickness: 1.6mm / Outer Copper: 1oz / Inner Copper: 0.5oz / Finish: HASL Lead Free / Red Solder Resist / White Silkscreen | Paul Clark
